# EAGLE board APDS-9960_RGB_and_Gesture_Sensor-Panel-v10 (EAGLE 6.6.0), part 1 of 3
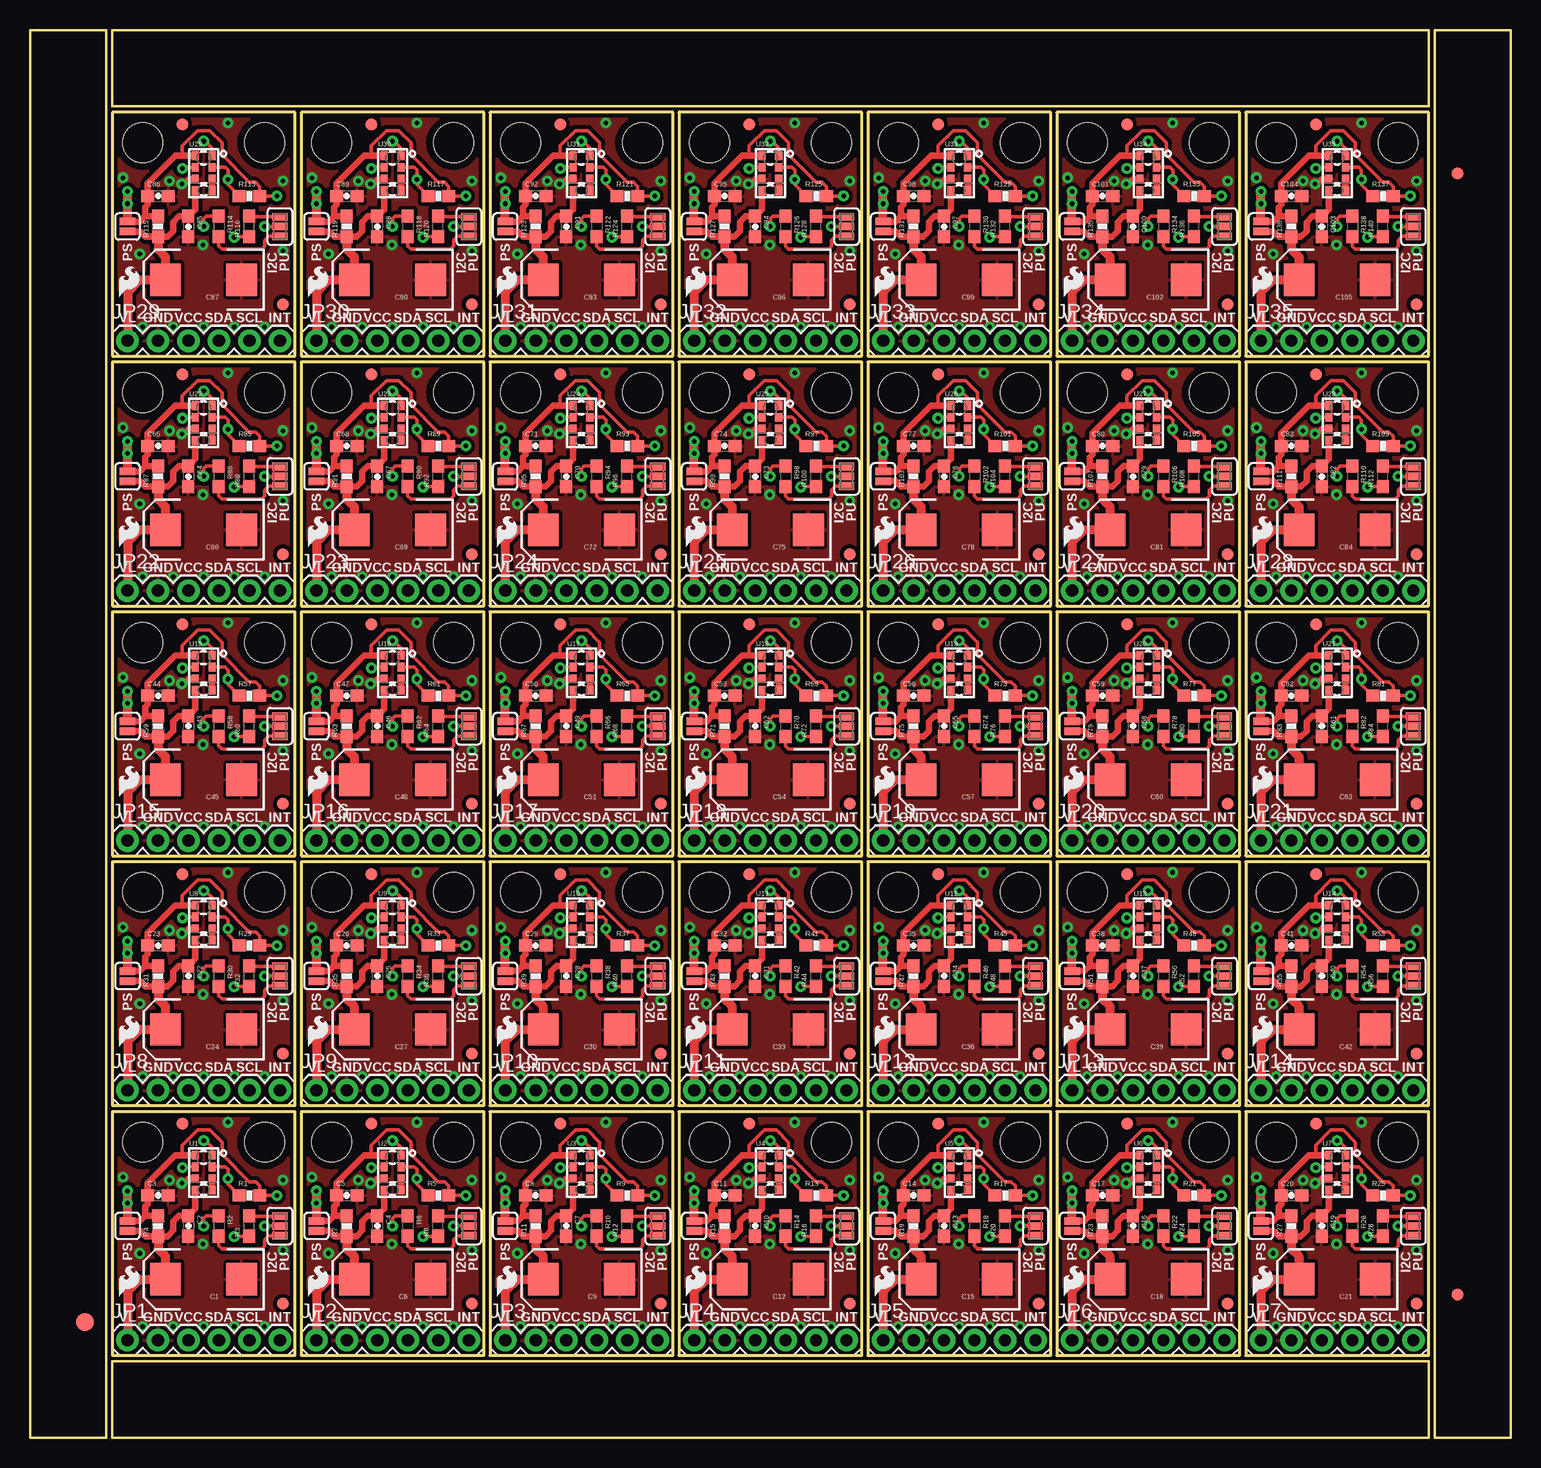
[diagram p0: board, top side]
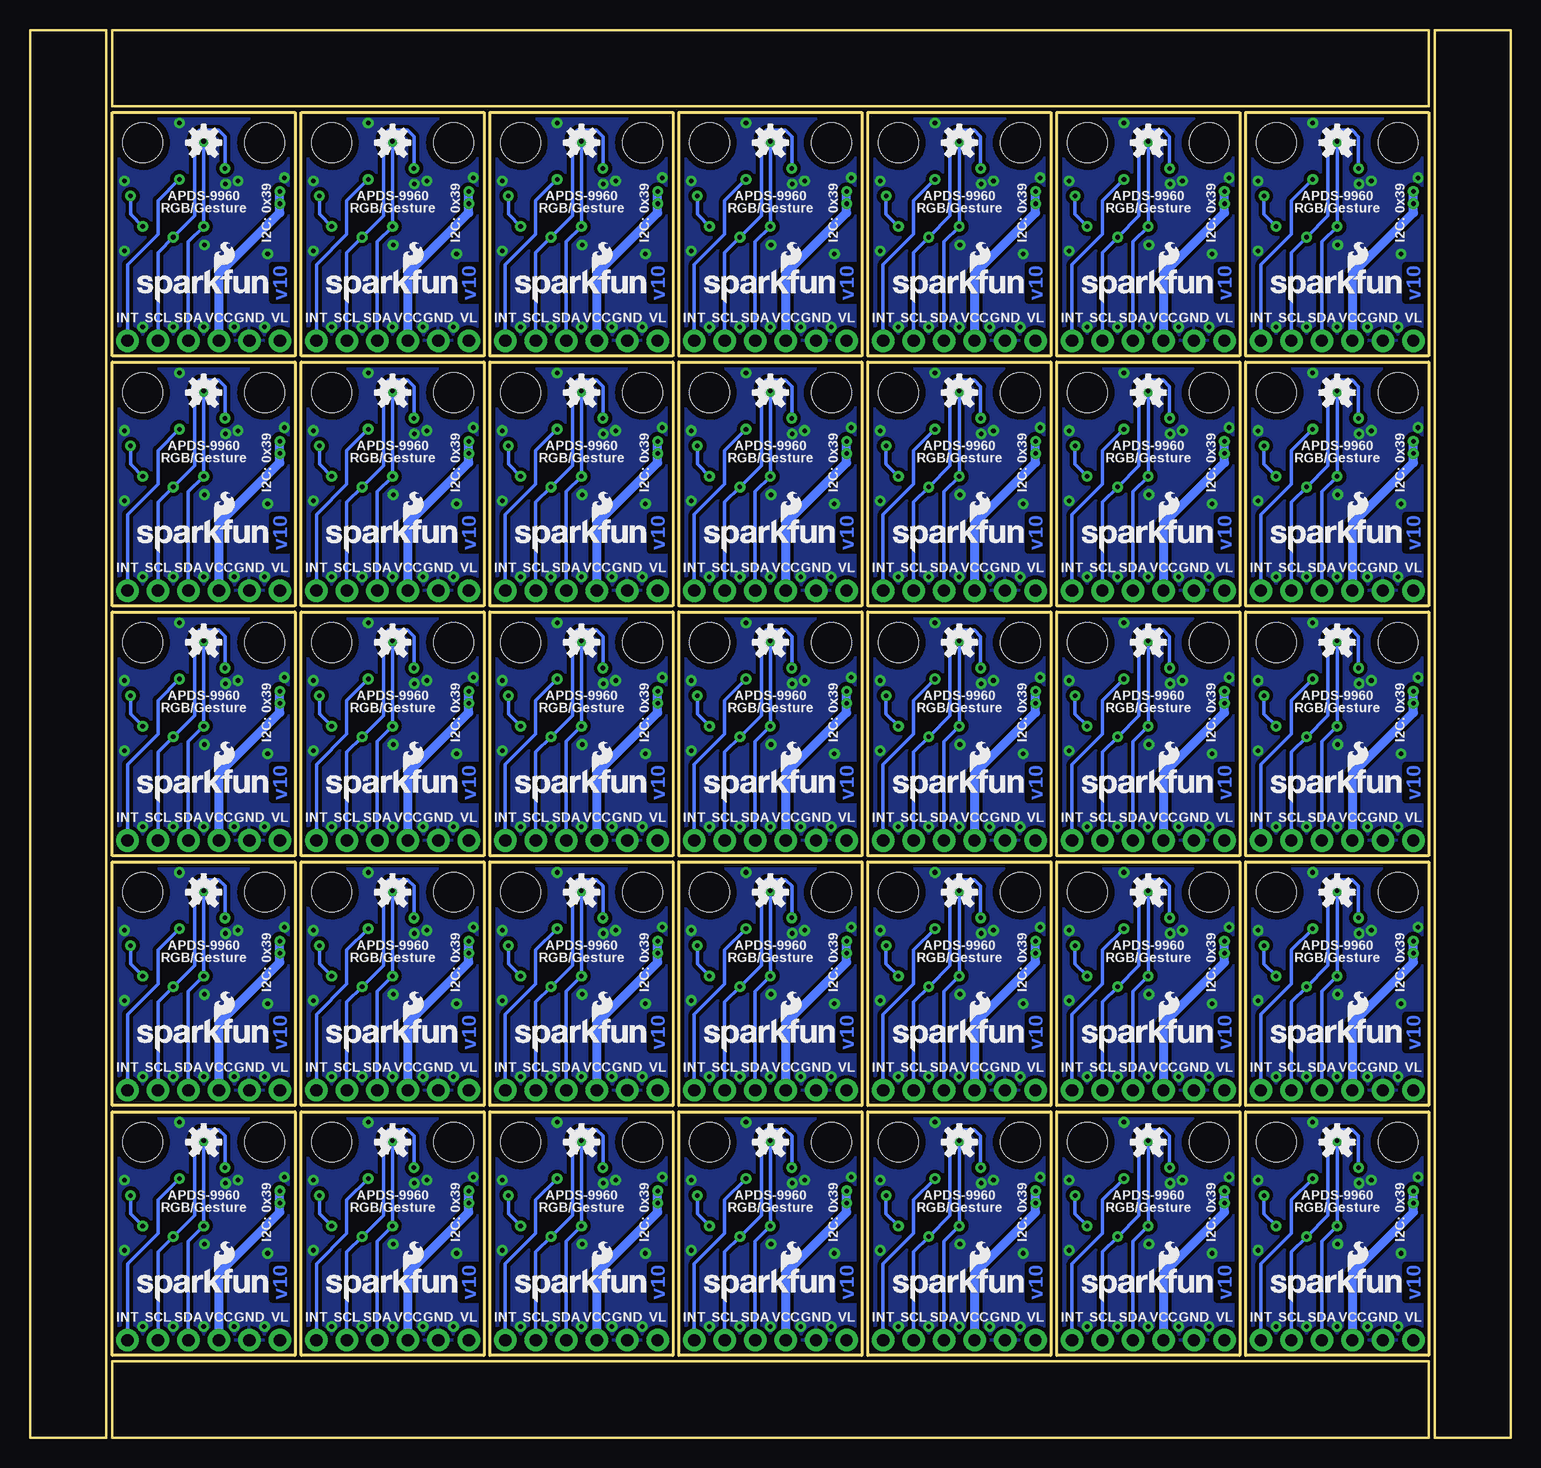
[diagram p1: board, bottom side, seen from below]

Size 123.44 x 117.35 mm. Coordinates in mm from the lower left corner, seen from the top.
Outline: 156 segments
Copper layers (1*16): Top 0.035mm / dielectric 1.5mm / Bottom 0.035mm
Design rules "SparkFun-2-layer": minimum track width 7mil, minimum drill 15mil, track to track 8mil, track to pad 8mil, pad to pad 8mil, via to via 8mil, smd to smd 8mil, copper to edge 8mil, drill to drill 8mil, minimum pad ring 12mil, minimum via ring 10mil, stop-mask expansion 4mil, vias tented up to drill 20mil, thermal gap 10mil

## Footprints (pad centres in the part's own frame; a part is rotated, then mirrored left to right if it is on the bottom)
EIA7343 = smd 2.55 x 2.7: A 3.17,0; C -3.17,0
0603-CAP = smd 1.1 x 1: 1 -0.85,0; 2 0.85,0
FIDUCIAL-1.5X3 = smd 1.5 x 1.5: 1 0,0
FIDUCIAL-1X2 = smd 1 x 1: 1 0,0
1X06 = drill 1.016 pad 1.88: 1 0,0; 2 2.54,0; 3 5.08,0; 4 7.62,0; 5 10.16,0; 6 12.7,0
0603-RES = smd 1.1 x 1: 1 -0.85,0; 2 0.85,0
0603 = smd 1.1 x 1: 1 -0.85,0; 2 0.85,0
SJ_3_PASTE1&2&3 = smd 0.635 x 1.27: 1 -0.813,0; 2 0,0; 3 0.813,0
SJ_2S = smd 0.635 x 1.27: 1 -0.412,0; 2 0.412,0
STAND-OFF = hole 3.302: 0,0
APDS-9960 = smd 0.6 x 0.72: 1 0.7,1.455; 2 0.7,0.485; 3 0.7,-0.485; 4 0.7,-1.455; 5 -0.7,-1.455; 6 -0.7,-0.485; 7 -0.7,0.485; 8 -0.7,1.455

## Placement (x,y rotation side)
C1  100uF  [EIA7343]  14.48,13.21 180 top
C2  1.0uF  [0603-CAP]  13.21,17.65 270 top
C3  1.0uF  [0603-CAP]  10.67,20.19 0 top
C4  1.0uF  [0603-CAP]  28.96,17.65 270 top
C5  1.0uF  [0603-CAP]  26.42,20.19 0 top
C6  100uF  [EIA7343]  30.23,13.21 180 top
C7  1.0uF  [0603-CAP]  44.7,17.65 270 top
C8  1.0uF  [0603-CAP]  42.16,20.19 0 top
C9  100uF  [EIA7343]  45.97,13.21 180 top
C10  1.0uF  [0603-CAP]  60.45,17.65 270 top
C11  1.0uF  [0603-CAP]  57.91,20.19 0 top
C12  100uF  [EIA7343]  61.72,13.21 180 top
C13  1.0uF  [0603-CAP]  76.2,17.65 270 top
C14  1.0uF  [0603-CAP]  73.66,20.19 0 top
C15  100uF  [EIA7343]  77.47,13.21 180 top
C16  1.0uF  [0603-CAP]  91.95,17.65 270 top
C17  1.0uF  [0603-CAP]  89.41,20.19 0 top
C18  100uF  [EIA7343]  93.22,13.21 180 top
C19  1.0uF  [0603-CAP]  107.7,17.65 270 top
C20  1.0uF  [0603-CAP]  105.16,20.19 0 top
C21  100uF  [EIA7343]  108.97,13.21 180 top
C22  1.0uF  [0603-CAP]  13.21,38.48 270 top
C23  1.0uF  [0603-CAP]  10.67,41.02 0 top
C24  100uF  [EIA7343]  14.48,34.04 180 top
C25  1.0uF  [0603-CAP]  28.96,38.48 270 top
C26  1.0uF  [0603-CAP]  26.42,41.02 0 top
C27  100uF  [EIA7343]  30.23,34.04 180 top
C28  1.0uF  [0603-CAP]  44.7,38.48 270 top
C29  1.0uF  [0603-CAP]  42.16,41.02 0 top
C30  100uF  [EIA7343]  45.97,34.04 180 top
C31  1.0uF  [0603-CAP]  60.45,38.48 270 top
C32  1.0uF  [0603-CAP]  57.91,41.02 0 top
C33  100uF  [EIA7343]  61.72,34.04 180 top
C34  1.0uF  [0603-CAP]  76.2,38.48 270 top
C35  1.0uF  [0603-CAP]  73.66,41.02 0 top
C36  100uF  [EIA7343]  77.47,34.04 180 top
C37  1.0uF  [0603-CAP]  91.95,38.48 270 top
C38  1.0uF  [0603-CAP]  89.41,41.02 0 top
C39  100uF  [EIA7343]  93.22,34.04 180 top
C40  1.0uF  [0603-CAP]  107.7,38.48 270 top
C41  1.0uF  [0603-CAP]  105.16,41.02 0 top
C42  100uF  [EIA7343]  108.97,34.04 180 top
C43  1.0uF  [0603-CAP]  13.21,59.31 270 top
C44  1.0uF  [0603-CAP]  10.67,61.85 0 top
C45  100uF  [EIA7343]  14.48,54.86 180 top
C46  1.0uF  [0603-CAP]  28.96,59.31 270 top
C47  1.0uF  [0603-CAP]  26.42,61.85 0 top
C48  100uF  [EIA7343]  30.23,54.86 180 top
C49  1.0uF  [0603-CAP]  44.7,59.31 270 top
C50  1.0uF  [0603-CAP]  42.16,61.85 0 top
C51  100uF  [EIA7343]  45.97,54.86 180 top
C52  1.0uF  [0603-CAP]  60.45,59.31 270 top
C53  1.0uF  [0603-CAP]  57.91,61.85 0 top
C54  100uF  [EIA7343]  61.72,54.86 180 top
C55  1.0uF  [0603-CAP]  76.2,59.31 270 top
C56  1.0uF  [0603-CAP]  73.66,61.85 0 top
C57  100uF  [EIA7343]  77.47,54.86 180 top
C58  1.0uF  [0603-CAP]  91.95,59.31 270 top
C59  1.0uF  [0603-CAP]  89.41,61.85 0 top
C60  100uF  [EIA7343]  93.22,54.86 180 top
C61  1.0uF  [0603-CAP]  107.7,59.31 270 top
C62  1.0uF  [0603-CAP]  105.16,61.85 0 top
C63  100uF  [EIA7343]  108.97,54.86 180 top
C64  1.0uF  [0603-CAP]  13.21,80.14 270 top
C65  1.0uF  [0603-CAP]  10.67,82.68 0 top
C66  100uF  [EIA7343]  14.48,75.69 180 top
C67  1.0uF  [0603-CAP]  28.96,80.14 270 top
C68  1.0uF  [0603-CAP]  26.42,82.68 0 top
C69  100uF  [EIA7343]  30.23,75.69 180 top
C70  1.0uF  [0603-CAP]  44.7,80.14 270 top
C71  1.0uF  [0603-CAP]  42.16,82.68 0 top
C72  100uF  [EIA7343]  45.97,75.69 180 top
C73  1.0uF  [0603-CAP]  60.45,80.14 270 top
C74  1.0uF  [0603-CAP]  57.91,82.68 0 top
C75  100uF  [EIA7343]  61.72,75.69 180 top
C76  1.0uF  [0603-CAP]  76.2,80.14 270 top
C77  1.0uF  [0603-CAP]  73.66,82.68 0 top
C78  100uF  [EIA7343]  77.47,75.69 180 top
C79  1.0uF  [0603-CAP]  91.95,80.14 270 top
C80  1.0uF  [0603-CAP]  89.41,82.68 0 top
C81  100uF  [EIA7343]  93.22,75.69 180 top
C82  1.0uF  [0603-CAP]  107.7,80.14 270 top
C83  1.0uF  [0603-CAP]  105.16,82.68 0 top
C84  100uF  [EIA7343]  108.97,75.69 180 top
C85  1.0uF  [0603-CAP]  13.21,100.97 270 top
C86  1.0uF  [0603-CAP]  10.67,103.5 0 top
C87  100uF  [EIA7343]  14.48,96.52 180 top
C88  1.0uF  [0603-CAP]  28.96,100.97 270 top
C89  1.0uF  [0603-CAP]  26.42,103.5 0 top
C90  100uF  [EIA7343]  30.23,96.52 180 top
C91  1.0uF  [0603-CAP]  44.7,100.97 270 top
C92  1.0uF  [0603-CAP]  42.16,103.5 0 top
C93  100uF  [EIA7343]  45.97,96.52 180 top
C94  1.0uF  [0603-CAP]  60.45,100.97 270 top
C95  1.0uF  [0603-CAP]  57.91,103.5 0 top
C96  100uF  [EIA7343]  61.72,96.52 180 top
C97  1.0uF  [0603-CAP]  76.2,100.97 270 top
C98  1.0uF  [0603-CAP]  73.66,103.5 0 top
C99  100uF  [EIA7343]  77.47,96.52 180 top
C100  1.0uF  [0603-CAP]  91.95,100.97 270 top
C101  1.0uF  [0603-CAP]  89.41,103.5 0 top
C102  100uF  [EIA7343]  93.22,96.52 180 top
C103  1.0uF  [0603-CAP]  107.7,100.97 270 top
C104  1.0uF  [0603-CAP]  105.16,103.5 0 top
C105  100uF  [EIA7343]  108.97,96.52 180 top
E$1  [FIDUCIAL-1.5X3]  4.57,9.65 0 top
E$4  [FIDUCIAL-1X2]  119,11.94 0 top
E$6  [FIDUCIAL-1X2]  119,105.41 180 top
FID1  FIDUCIAL1X2  [FIDUCIAL-1X2]  21.08,11.18 0 top
FID2  FIDUCIAL1X2  [FIDUCIAL-1X2]  12.7,26.16 0 top
FID3  FIDUCIAL1X2  [FIDUCIAL-1X2]  36.83,11.18 0 top
FID4  FIDUCIAL1X2  [FIDUCIAL-1X2]  28.45,26.16 0 top
FID5  FIDUCIAL1X2  [FIDUCIAL-1X2]  52.58,11.18 0 top
FID6  FIDUCIAL1X2  [FIDUCIAL-1X2]  44.2,26.16 0 top
FID7  FIDUCIAL1X2  [FIDUCIAL-1X2]  68.33,11.18 0 top
FID8  FIDUCIAL1X2  [FIDUCIAL-1X2]  59.94,26.16 0 top
FID9  FIDUCIAL1X2  [FIDUCIAL-1X2]  84.07,11.18 0 top
FID10  FIDUCIAL1X2  [FIDUCIAL-1X2]  75.69,26.16 0 top
FID11  FIDUCIAL1X2  [FIDUCIAL-1X2]  99.82,11.18 0 top
FID12  FIDUCIAL1X2  [FIDUCIAL-1X2]  91.44,26.16 0 top
FID13  FIDUCIAL1X2  [FIDUCIAL-1X2]  115.57,11.18 0 top
FID14  FIDUCIAL1X2  [FIDUCIAL-1X2]  107.19,26.16 0 top
FID15  FIDUCIAL1X2  [FIDUCIAL-1X2]  21.08,32 0 top
FID16  FIDUCIAL1X2  [FIDUCIAL-1X2]  12.7,46.99 0 top
FID17  FIDUCIAL1X2  [FIDUCIAL-1X2]  36.83,32 0 top
FID18  FIDUCIAL1X2  [FIDUCIAL-1X2]  28.45,46.99 0 top
FID19  FIDUCIAL1X2  [FIDUCIAL-1X2]  52.58,32 0 top
FID20  FIDUCIAL1X2  [FIDUCIAL-1X2]  44.2,46.99 0 top
FID21  FIDUCIAL1X2  [FIDUCIAL-1X2]  68.33,32 0 top
FID22  FIDUCIAL1X2  [FIDUCIAL-1X2]  59.94,46.99 0 top
FID23  FIDUCIAL1X2  [FIDUCIAL-1X2]  84.07,32 0 top
FID24  FIDUCIAL1X2  [FIDUCIAL-1X2]  75.69,46.99 0 top
FID25  FIDUCIAL1X2  [FIDUCIAL-1X2]  99.82,32 0 top
FID26  FIDUCIAL1X2  [FIDUCIAL-1X2]  91.44,46.99 0 top
FID27  FIDUCIAL1X2  [FIDUCIAL-1X2]  115.57,32 0 top
FID28  FIDUCIAL1X2  [FIDUCIAL-1X2]  107.19,46.99 0 top
FID29  FIDUCIAL1X2  [FIDUCIAL-1X2]  21.08,52.83 0 top
FID30  FIDUCIAL1X2  [FIDUCIAL-1X2]  12.7,67.82 0 top
FID31  FIDUCIAL1X2  [FIDUCIAL-1X2]  36.83,52.83 0 top
FID32  FIDUCIAL1X2  [FIDUCIAL-1X2]  28.45,67.82 0 top
FID33  FIDUCIAL1X2  [FIDUCIAL-1X2]  52.58,52.83 0 top
FID34  FIDUCIAL1X2  [FIDUCIAL-1X2]  44.2,67.82 0 top
FID35  FIDUCIAL1X2  [FIDUCIAL-1X2]  68.33,52.83 0 top
FID36  FIDUCIAL1X2  [FIDUCIAL-1X2]  59.94,67.82 0 top
FID37  FIDUCIAL1X2  [FIDUCIAL-1X2]  84.07,52.83 0 top
FID38  FIDUCIAL1X2  [FIDUCIAL-1X2]  75.69,67.82 0 top
FID39  FIDUCIAL1X2  [FIDUCIAL-1X2]  99.82,52.83 0 top
FID40  FIDUCIAL1X2  [FIDUCIAL-1X2]  91.44,67.82 0 top
FID41  FIDUCIAL1X2  [FIDUCIAL-1X2]  115.57,52.83 0 top
FID42  FIDUCIAL1X2  [FIDUCIAL-1X2]  107.19,67.82 0 top
FID43  FIDUCIAL1X2  [FIDUCIAL-1X2]  21.08,73.66 0 top
FID44  FIDUCIAL1X2  [FIDUCIAL-1X2]  12.7,88.65 0 top
FID45  FIDUCIAL1X2  [FIDUCIAL-1X2]  36.83,73.66 0 top
FID46  FIDUCIAL1X2  [FIDUCIAL-1X2]  28.45,88.65 0 top
FID47  FIDUCIAL1X2  [FIDUCIAL-1X2]  52.58,73.66 0 top
FID48  FIDUCIAL1X2  [FIDUCIAL-1X2]  44.2,88.65 0 top
FID49  FIDUCIAL1X2  [FIDUCIAL-1X2]  68.33,73.66 0 top
FID50  FIDUCIAL1X2  [FIDUCIAL-1X2]  59.94,88.65 0 top
FID51  FIDUCIAL1X2  [FIDUCIAL-1X2]  84.07,73.66 0 top
FID52  FIDUCIAL1X2  [FIDUCIAL-1X2]  75.69,88.65 0 top
FID53  FIDUCIAL1X2  [FIDUCIAL-1X2]  99.82,73.66 0 top
FID54  FIDUCIAL1X2  [FIDUCIAL-1X2]  91.44,88.65 0 top
FID55  FIDUCIAL1X2  [FIDUCIAL-1X2]  115.57,73.66 0 top
FID56  FIDUCIAL1X2  [FIDUCIAL-1X2]  107.19,88.65 0 top
FID57  FIDUCIAL1X2  [FIDUCIAL-1X2]  21.08,94.49 0 top
FID58  FIDUCIAL1X2  [FIDUCIAL-1X2]  12.7,109.47 0 top
FID59  FIDUCIAL1X2  [FIDUCIAL-1X2]  36.83,94.49 0 top
FID60  FIDUCIAL1X2  [FIDUCIAL-1X2]  28.45,109.47 0 top
FID61  FIDUCIAL1X2  [FIDUCIAL-1X2]  52.58,94.49 0 top
FID62  FIDUCIAL1X2  [FIDUCIAL-1X2]  44.2,109.47 0 top
FID63  FIDUCIAL1X2  [FIDUCIAL-1X2]  68.33,94.49 0 top
FID64  FIDUCIAL1X2  [FIDUCIAL-1X2]  59.94,109.47 0 top
FID65  FIDUCIAL1X2  [FIDUCIAL-1X2]  84.07,94.49 0 top
FID66  FIDUCIAL1X2  [FIDUCIAL-1X2]  75.69,109.47 0 top
FID67  FIDUCIAL1X2  [FIDUCIAL-1X2]  99.82,94.49 0 top
FID68  FIDUCIAL1X2  [FIDUCIAL-1X2]  91.44,109.47 0 top
FID69  FIDUCIAL1X2  [FIDUCIAL-1X2]  115.57,94.49 0 top
FID70  FIDUCIAL1X2  [FIDUCIAL-1X2]  107.19,109.47 0 top
JP1  [1X06]  8.13,8.13 0 top
JP2  [1X06]  23.88,8.13 0 top
JP3  [1X06]  39.62,8.13 0 top
JP4  [1X06]  55.37,8.13 0 top
JP5  [1X06]  71.12,8.13 0 top
JP6  [1X06]  86.87,8.13 0 top
JP7  [1X06]  102.62,8.13 0 top
JP8  [1X06]  8.13,28.96 0 top
JP9  [1X06]  23.88,28.96 0 top
JP10  [1X06]  39.62,28.96 0 top
JP11  [1X06]  55.37,28.96 0 top
JP12  [1X06]  71.12,28.96 0 top
JP13  [1X06]  86.87,28.96 0 top
JP14  [1X06]  102.62,28.96 0 top
JP15  [1X06]  8.13,49.78 0 top
JP16  [1X06]  23.88,49.78 0 top
JP17  [1X06]  39.62,49.78 0 top
JP18  [1X06]  55.37,49.78 0 top
JP19  [1X06]  71.12,49.78 0 top
JP20  [1X06]  86.87,49.78 0 top
JP21  [1X06]  102.62,49.78 0 top
JP22  [1X06]  8.13,70.61 0 top
JP23  [1X06]  23.88,70.61 0 top
JP24  [1X06]  39.62,70.61 0 top
JP25  [1X06]  55.37,70.61 0 top
JP26  [1X06]  71.12,70.61 0 top
JP27  [1X06]  86.87,70.61 0 top
JP28  [1X06]  102.62,70.61 0 top
JP29  [1X06]  8.13,91.44 0 top
JP30  [1X06]  23.88,91.44 0 top
JP31  [1X06]  39.62,91.44 0 top
JP32  [1X06]  55.37,91.44 0 top
JP33  [1X06]  71.12,91.44 0 top
JP34  [1X06]  86.87,91.44 0 top
JP35  [1X06]  102.62,91.44 0 top
LOGO1  SFE_LOGO_FLAME.1_INCH  [SFE_LOGO_FLAME_.1]  7.11,11.43 0 top
LOGO2  OSHW-LOGOS  [OSHW-LOGO-S]  14.48,24.64 0 bottom
LOGO3  SFE_LOGO_FLAME.1_INCH  [SFE_LOGO_FLAME_.1]  22.86,11.43 0 top
LOGO4  OSHW-LOGOS  [OSHW-LOGO-S]  30.23,24.64 0 bottom
LOGO5  SFE_LOGO_FLAME.1_INCH  [SFE_LOGO_FLAME_.1]  38.61,11.43 0 top
LOGO6  OSHW-LOGOS  [OSHW-LOGO-S]  45.97,24.64 0 bottom
LOGO7  SFE_LOGO_FLAME.1_INCH  [SFE_LOGO_FLAME_.1]  54.36,11.43 0 top
LOGO8  OSHW-LOGOS  [OSHW-LOGO-S]  61.72,24.64 0 bottom
LOGO9  SFE_LOGO_FLAME.1_INCH  [SFE_LOGO_FLAME_.1]  70.1,11.43 0 top
LOGO10  OSHW-LOGOS  [OSHW-LOGO-S]  77.47,24.64 0 bottom
LOGO11  SFE_LOGO_FLAME.1_INCH  [SFE_LOGO_FLAME_.1]  85.85,11.43 0 top
LOGO12  OSHW-LOGOS  [OSHW-LOGO-S]  93.22,24.64 0 bottom
LOGO13  SFE_LOGO_FLAME.1_INCH  [SFE_LOGO_FLAME_.1]  101.6,11.43 0 top
LOGO14  OSHW-LOGOS  [OSHW-LOGO-S]  108.97,24.64 0 bottom
LOGO15  SFE_LOGO_FLAME.1_INCH  [SFE_LOGO_FLAME_.1]  7.11,32.26 0 top
LOGO16  OSHW-LOGOS  [OSHW-LOGO-S]  14.48,45.47 0 bottom
LOGO17  SFE_LOGO_FLAME.1_INCH  [SFE_LOGO_FLAME_.1]  22.86,32.26 0 top
LOGO18  OSHW-LOGOS  [OSHW-LOGO-S]  30.23,45.47 0 bottom
LOGO19  SFE_LOGO_FLAME.1_INCH  [SFE_LOGO_FLAME_.1]  38.61,32.26 0 top
LOGO20  OSHW-LOGOS  [OSHW-LOGO-S]  45.97,45.47 0 bottom
LOGO21  SFE_LOGO_FLAME.1_INCH  [SFE_LOGO_FLAME_.1]  54.36,32.26 0 top
LOGO22  OSHW-LOGOS  [OSHW-LOGO-S]  61.72,45.47 0 bottom
LOGO23  SFE_LOGO_FLAME.1_INCH  [SFE_LOGO_FLAME_.1]  70.1,32.26 0 top
LOGO24  OSHW-LOGOS  [OSHW-LOGO-S]  77.47,45.47 0 bottom
LOGO25  SFE_LOGO_FLAME.1_INCH  [SFE_LOGO_FLAME_.1]  85.85,32.26 0 top
LOGO26  OSHW-LOGOS  [OSHW-LOGO-S]  93.22,45.47 0 bottom
LOGO27  SFE_LOGO_FLAME.1_INCH  [SFE_LOGO_FLAME_.1]  101.6,32.26 0 top
LOGO28  OSHW-LOGOS  [OSHW-LOGO-S]  108.97,45.47 0 bottom
LOGO29  SFE_LOGO_FLAME.1_INCH  [SFE_LOGO_FLAME_.1]  7.11,53.09 0 top
LOGO30  OSHW-LOGOS  [OSHW-LOGO-S]  14.48,66.29 0 bottom
LOGO31  SFE_LOGO_FLAME.1_INCH  [SFE_LOGO_FLAME_.1]  22.86,53.09 0 top
LOGO32  OSHW-LOGOS  [OSHW-LOGO-S]  30.23,66.29 0 bottom
LOGO33  SFE_LOGO_FLAME.1_INCH  [SFE_LOGO_FLAME_.1]  38.61,53.09 0 top
LOGO34  OSHW-LOGOS  [OSHW-LOGO-S]  45.97,66.29 0 bottom
LOGO35  SFE_LOGO_FLAME.1_INCH  [SFE_LOGO_FLAME_.1]  54.36,53.09 0 top
LOGO36  OSHW-LOGOS  [OSHW-LOGO-S]  61.72,66.29 0 bottom
LOGO37  SFE_LOGO_FLAME.1_INCH  [SFE_LOGO_FLAME_.1]  70.1,53.09 0 top
LOGO38  OSHW-LOGOS  [OSHW-LOGO-S]  77.47,66.29 0 bottom
LOGO39  SFE_LOGO_FLAME.1_INCH  [SFE_LOGO_FLAME_.1]  85.85,53.09 0 top
LOGO40  OSHW-LOGOS  [OSHW-LOGO-S]  93.22,66.29 0 bottom
LOGO41  SFE_LOGO_FLAME.1_INCH  [SFE_LOGO_FLAME_.1]  101.6,53.09 0 top
LOGO42  OSHW-LOGOS  [OSHW-LOGO-S]  108.97,66.29 0 bottom
LOGO43  SFE_LOGO_FLAME.1_INCH  [SFE_LOGO_FLAME_.1]  7.11,73.91 0 top
LOGO44  OSHW-LOGOS  [OSHW-LOGO-S]  14.48,87.12 0 bottom
LOGO45  SFE_LOGO_FLAME.1_INCH  [SFE_LOGO_FLAME_.1]  22.86,73.91 0 top
LOGO46  OSHW-LOGOS  [OSHW-LOGO-S]  30.23,87.12 0 bottom
LOGO47  SFE_LOGO_FLAME.1_INCH  [SFE_LOGO_FLAME_.1]  38.61,73.91 0 top
LOGO48  OSHW-LOGOS  [OSHW-LOGO-S]  45.97,87.12 0 bottom
LOGO49  SFE_LOGO_FLAME.1_INCH  [SFE_LOGO_FLAME_.1]  54.36,73.91 0 top
LOGO50  OSHW-LOGOS  [OSHW-LOGO-S]  61.72,87.12 0 bottom
LOGO51  SFE_LOGO_FLAME.1_INCH  [SFE_LOGO_FLAME_.1]  70.1,73.91 0 top
LOGO52  OSHW-LOGOS  [OSHW-LOGO-S]  77.47,87.12 0 bottom
LOGO53  SFE_LOGO_FLAME.1_INCH  [SFE_LOGO_FLAME_.1]  85.85,73.91 0 top
LOGO54  OSHW-LOGOS  [OSHW-LOGO-S]  93.22,87.12 0 bottom
LOGO55  SFE_LOGO_FLAME.1_INCH  [SFE_LOGO_FLAME_.1]  101.6,73.91 0 top
LOGO56  OSHW-LOGOS  [OSHW-LOGO-S]  108.97,87.12 0 bottom
LOGO57  SFE_LOGO_FLAME.1_INCH  [SFE_LOGO_FLAME_.1]  7.11,94.74 0 top
LOGO58  OSHW-LOGOS  [OSHW-LOGO-S]  14.48,107.95 0 bottom
LOGO59  SFE_LOGO_FLAME.1_INCH  [SFE_LOGO_FLAME_.1]  22.86,94.74 0 top
LOGO60  OSHW-LOGOS  [OSHW-LOGO-S]  30.23,107.95 0 bottom
LOGO61  SFE_LOGO_FLAME.1_INCH  [SFE_LOGO_FLAME_.1]  38.61,94.74 0 top
LOGO62  OSHW-LOGOS  [OSHW-LOGO-S]  45.97,107.95 0 bottom
LOGO63  SFE_LOGO_FLAME.1_INCH  [SFE_LOGO_FLAME_.1]  54.36,94.74 0 top
LOGO64  OSHW-LOGOS  [OSHW-LOGO-S]  61.72,107.95 0 bottom
LOGO65  SFE_LOGO_FLAME.1_INCH  [SFE_LOGO_FLAME_.1]  70.1,94.74 0 top
LOGO66  OSHW-LOGOS  [OSHW-LOGO-S]  77.47,107.95 0 bottom
LOGO67  SFE_LOGO_FLAME.1_INCH  [SFE_LOGO_FLAME_.1]  85.85,94.74 0 top
LOGO68  OSHW-LOGOS  [OSHW-LOGO-S]  93.22,107.95 0 bottom
LOGO69  SFE_LOGO_FLAME.1_INCH  [SFE_LOGO_FLAME_.1]  101.6,94.74 0 top
LOGO70  OSHW-LOGOS  [OSHW-LOGO-S]  108.97,107.95 0 bottom
R1  10k  [0603-RES]  18.29,20.19 0 top
R2  4.7k  [0603]  15.75,17.65 270 top
R3  4.7k  [0603]  18.29,17.65 90 top
R4  DNP  [0603-RES]  10.67,17.65 90 top
R5  10k  [0603-RES]  34.04,20.19 0 top
R6  4.7k  [0603]  31.5,17.65 270 top
R7  DNP  [0603-RES]  26.42,17.65 90 top
R8  4.7k  [0603]  34.04,17.65 90 top
R9  10k  [0603-RES]  49.78,20.19 0 top
R10  4.7k  [0603]  47.24,17.65 270 top
R11  DNP  [0603-RES]  42.16,17.65 90 top
R12  4.7k  [0603]  49.78,17.65 90 top
R13  10k  [0603-RES]  65.53,20.19 0 top
R14  4.7k  [0603]  62.99,17.65 270 top
R15  DNP  [0603-RES]  57.91,17.65 90 top
R16  4.7k  [0603]  65.53,17.65 90 top
R17  10k  [0603-RES]  81.28,20.19 0 top
R18  4.7k  [0603]  78.74,17.65 270 top
R19  DNP  [0603-RES]  73.66,17.65 90 top
R20  4.7k  [0603]  81.28,17.65 90 top
R21  10k  [0603-RES]  97.03,20.19 0 top
R22  4.7k  [0603]  94.49,17.65 270 top
R23  DNP  [0603-RES]  89.41,17.65 90 top
R24  4.7k  [0603]  97.03,17.65 90 top
R25  10k  [0603-RES]  112.78,20.19 0 top
R26  4.7k  [0603]  110.24,17.65 270 top
R27  DNP  [0603-RES]  105.16,17.65 90 top
R28  4.7k  [0603]  112.78,17.65 90 top
R29  10k  [0603-RES]  18.29,41.02 0 top
R30  4.7k  [0603]  15.75,38.48 270 top
R31  DNP  [0603-RES]  10.67,38.48 90 top
R32  4.7k  [0603]  18.29,38.48 90 top
R33  10k  [0603-RES]  34.04,41.02 0 top
R34  4.7k  [0603]  31.5,38.48 270 top
R35  DNP  [0603-RES]  26.42,38.48 90 top
R36  4.7k  [0603]  34.04,38.48 90 top
R37  10k  [0603-RES]  49.78,41.02 0 top
R38  4.7k  [0603]  47.24,38.48 270 top
R39  DNP  [0603-RES]  42.16,38.48 90 top
R40  4.7k  [0603]  49.78,38.48 90 top
R41  10k  [0603-RES]  65.53,41.02 0 top
R42  4.7k  [0603]  62.99,38.48 270 top
R43  DNP  [0603-RES]  57.91,38.48 90 top
R44  4.7k  [0603]  65.53,38.48 90 top
R45  10k  [0603-RES]  81.28,41.02 0 top
R46  4.7k  [0603]  78.74,38.48 270 top
R47  DNP  [0603-RES]  73.66,38.48 90 top
R48  4.7k  [0603]  81.28,38.48 90 top
R49  10k  [0603-RES]  97.03,41.02 0 top
R50  4.7k  [0603]  94.49,38.48 270 top
R51  DNP  [0603-RES]  89.41,38.48 90 top
R52  4.7k  [0603]  97.03,38.48 90 top
R53  10k  [0603-RES]  112.78,41.02 0 top
R54  4.7k  [0603]  110.24,38.48 270 top
R55  DNP  [0603-RES]  105.16,38.48 90 top
R56  4.7k  [0603]  112.78,38.48 90 top
R57  10k  [0603-RES]  18.29,61.85 0 top
R58  4.7k  [0603]  15.75,59.31 270 top
R59  DNP  [0603-RES]  10.67,59.31 90 top
R60  4.7k  [0603]  18.29,59.31 90 top
R61  10k  [0603-RES]  34.04,61.85 0 top
R62  4.7k  [0603]  31.5,59.31 270 top
R63  DNP  [0603-RES]  26.42,59.31 90 top
R64  4.7k  [0603]  34.04,59.31 90 top
R65  10k  [0603-RES]  49.78,61.85 0 top
R66  4.7k  [0603]  47.24,59.31 270 top
R67  DNP  [0603-RES]  42.16,59.31 90 top
R68  4.7k  [0603]  49.78,59.31 90 top
R69  10k  [0603-RES]  65.53,61.85 0 top
R70  4.7k  [0603]  62.99,59.31 270 top
R71  DNP  [0603-RES]  57.91,59.31 90 top
R72  4.7k  [0603]  65.53,59.31 90 top
R73  10k  [0603-RES]  81.28,61.85 0 top
R74  4.7k  [0603]  78.74,59.31 270 top
R75  DNP  [0603-RES]  73.66,59.31 90 top
R76  4.7k  [0603]  81.28,59.31 90 top
R77  10k  [0603-RES]  97.03,61.85 0 top
R78  4.7k  [0603]  94.49,59.31 270 top
R79  DNP  [0603-RES]  89.41,59.31 90 top
R80  4.7k  [0603]  97.03,59.31 90 top
R81  10k  [0603-RES]  112.78,61.85 0 top
R82  4.7k  [0603]  110.24,59.31 270 top
R83  DNP  [0603-RES]  105.16,59.31 90 top
R84  4.7k  [0603]  112.78,59.31 90 top
R85  10k  [0603-RES]  18.29,82.68 0 top
R86  4.7k  [0603]  15.75,80.14 270 top
R87  DNP  [0603-RES]  10.67,80.14 90 top
R88  4.7k  [0603]  18.29,80.14 90 top
R89  10k  [0603-RES]  34.04,82.68 0 top
R90  4.7k  [0603]  31.5,80.14 270 top
R91  DNP  [0603-RES]  26.42,80.14 90 top
R92  4.7k  [0603]  34.04,80.14 90 top
R93  10k  [0603-RES]  49.78,82.68 0 top
R94  4.7k  [0603]  47.24,80.14 270 top
R95  DNP  [0603-RES]  42.16,80.14 90 top
R96  4.7k  [0603]  49.78,80.14 90 top
R97  10k  [0603-RES]  65.53,82.68 0 top
R98  4.7k  [0603]  62.99,80.14 270 top
R99  DNP  [0603-RES]  57.91,80.14 90 top
R100  4.7k  [0603]  65.53,80.14 90 top
R101  10k  [0603-RES]  81.28,82.68 0 top
R102  4.7k  [0603]  78.74,80.14 270 top
R103  DNP  [0603-RES]  73.66,80.14 90 top
R104  4.7k  [0603]  81.28,80.14 90 top
R105  10k  [0603-RES]  97.03,82.68 0 top
R106  4.7k  [0603]  94.49,80.14 270 top
R107  DNP  [0603-RES]  89.41,80.14 90 top
R108  4.7k  [0603]  97.03,80.14 90 top
R109  10k  [0603-RES]  112.78,82.68 0 top
R110  4.7k  [0603]  110.24,80.14 270 top
R111  DNP  [0603-RES]  105.16,80.14 90 top
R112  4.7k  [0603]  112.78,80.14 90 top
R113  10k  [0603-RES]  18.29,103.5 0 top
R114  4.7k  [0603]  15.75,100.97 270 top
R115  DNP  [0603-RES]  10.67,100.97 90 top
R116  4.7k  [0603]  18.29,100.97 90 top
R117  10k  [0603-RES]  34.04,103.5 0 top
R118  4.7k  [0603]  31.5,100.97 270 top
R119  DNP  [0603-RES]  26.42,100.97 90 top
R120  4.7k  [0603]  34.04,100.97 90 top
R121  10k  [0603-RES]  49.78,103.5 0 top
R122  4.7k  [0603]  47.24,100.97 270 top
R123  DNP  [0603-RES]  42.16,100.97 90 top
R124  4.7k  [0603]  49.78,100.97 90 top
R125  10k  [0603-RES]  65.53,103.5 0 top
R126  4.7k  [0603]  62.99,100.97 270 top
R127  DNP  [0603-RES]  57.91,100.97 90 top
R128  4.7k  [0603]  65.53,100.97 90 top
R129  10k  [0603-RES]  81.28,103.5 0 top
R130  4.7k  [0603]  78.74,100.97 270 top
R131  DNP  [0603-RES]  73.66,100.97 90 top
R132  4.7k  [0603]  81.28,100.97 90 top
R133  10k  [0603-RES]  97.03,103.5 0 top
R134  4.7k  [0603]  94.49,100.97 270 top
R135  DNP  [0603-RES]  89.41,100.97 90 top
R136  4.7k  [0603]  97.03,100.97 90 top
R137  10k  [0603-RES]  112.78,103.5 0 top
R138  4.7k  [0603]  110.24,100.97 270 top
R139  DNP  [0603-RES]  105.16,100.97 90 top
R140  4.7k  [0603]  112.78,100.97 90 top
SJ1  [SJ_3_PASTE1&2&3]  20.83,17.65 270 top
SJ2  SOLDERJUMPERNC  [SJ_2S]  8.13,17.65 90 top
SJ3  [SJ_3_PASTE1&2&3]  36.58,17.65 270 top
SJ4  SOLDERJUMPERNC  [SJ_2S]  23.88,17.65 90 top
SJ5  [SJ_3_PASTE1&2&3]  52.32,17.65 270 top
SJ6  SOLDERJUMPERNC  [SJ_2S]  39.62,17.65 90 top
SJ7  [SJ_3_PASTE1&2&3]  68.07,17.65 270 top
SJ8  SOLDERJUMPERNC  [SJ_2S]  55.37,17.65 90 top
SJ9  [SJ_3_PASTE1&2&3]  83.82,17.65 270 top
SJ10  SOLDERJUMPERNC  [SJ_2S]  71.12,17.65 90 top
SJ11  [SJ_3_PASTE1&2&3]  99.57,17.65 270 top
SJ12  SOLDERJUMPERNC  [SJ_2S]  86.87,17.65 90 top
SJ13  [SJ_3_PASTE1&2&3]  115.32,17.65 270 top
SJ14  SOLDERJUMPERNC  [SJ_2S]  102.62,17.65 90 top
SJ15  [SJ_3_PASTE1&2&3]  20.83,38.48 270 top
SJ16  SOLDERJUMPERNC  [SJ_2S]  8.13,38.48 90 top
SJ17  [SJ_3_PASTE1&2&3]  36.58,38.48 270 top
SJ18  SOLDERJUMPERNC  [SJ_2S]  23.88,38.48 90 top
SJ19  [SJ_3_PASTE1&2&3]  52.32,38.48 270 top
SJ20  SOLDERJUMPERNC  [SJ_2S]  39.62,38.48 90 top
SJ21  [SJ_3_PASTE1&2&3]  68.07,38.48 270 top
SJ22  SOLDERJUMPERNC  [SJ_2S]  55.37,38.48 90 top
SJ23  [SJ_3_PASTE1&2&3]  83.82,38.48 270 top
SJ24  SOLDERJUMPERNC  [SJ_2S]  71.12,38.48 90 top
SJ25  [SJ_3_PASTE1&2&3]  99.57,38.48 270 top
SJ26  SOLDERJUMPERNC  [SJ_2S]  86.87,38.48 90 top
SJ27  [SJ_3_PASTE1&2&3]  115.32,38.48 270 top
SJ28  SOLDERJUMPERNC  [SJ_2S]  102.62,38.48 90 top
SJ29  [SJ_3_PASTE1&2&3]  20.83,59.31 270 top
SJ30  SOLDERJUMPERNC  [SJ_2S]  8.13,59.31 90 top
SJ31  [SJ_3_PASTE1&2&3]  36.58,59.31 270 top
SJ32  SOLDERJUMPERNC  [SJ_2S]  23.88,59.31 90 top
SJ33  [SJ_3_PASTE1&2&3]  52.32,59.31 270 top
SJ34  SOLDERJUMPERNC  [SJ_2S]  39.62,59.31 90 top
SJ35  [SJ_3_PASTE1&2&3]  68.07,59.31 270 top
SJ36  SOLDERJUMPERNC  [SJ_2S]  55.37,59.31 90 top
SJ37  [SJ_3_PASTE1&2&3]  83.82,59.31 270 top
SJ38  SOLDERJUMPERNC  [SJ_2S]  71.12,59.31 90 top
SJ39  [SJ_3_PASTE1&2&3]  99.57,59.31 270 top
SJ40  SOLDERJUMPERNC  [SJ_2S]  86.87,59.31 90 top
SJ41  [SJ_3_PASTE1&2&3]  115.32,59.31 270 top
SJ42  SOLDERJUMPERNC  [SJ_2S]  102.62,59.31 90 top
SJ43  [SJ_3_PASTE1&2&3]  20.83,80.14 270 top
SJ44  SOLDERJUMPERNC  [SJ_2S]  8.13,80.14 90 top
SJ45  [SJ_3_PASTE1&2&3]  36.58,80.14 270 top
SJ46  SOLDERJUMPERNC  [SJ_2S]  23.88,80.14 90 top
SJ47  [SJ_3_PASTE1&2&3]  52.32,80.14 270 top
SJ48  SOLDERJUMPERNC  [SJ_2S]  39.62,80.14 90 top
SJ49  [SJ_3_PASTE1&2&3]  68.07,80.14 270 top
SJ50  SOLDERJUMPERNC  [SJ_2S]  55.37,80.14 90 top
SJ51  [SJ_3_PASTE1&2&3]  83.82,80.14 270 top
SJ52  SOLDERJUMPERNC  [SJ_2S]  71.12,80.14 90 top
SJ53  [SJ_3_PASTE1&2&3]  99.57,80.14 270 top
SJ54  SOLDERJUMPERNC  [SJ_2S]  86.87,80.14 90 top
SJ55  [SJ_3_PASTE1&2&3]  115.32,80.14 270 top
SJ56  SOLDERJUMPERNC  [SJ_2S]  102.62,80.14 90 top
SJ57  [SJ_3_PASTE1&2&3]  20.83,100.97 270 top
SJ58  SOLDERJUMPERNC  [SJ_2S]  8.13,100.97 90 top
SJ59  [SJ_3_PASTE1&2&3]  36.58,100.97 270 top
SJ60  SOLDERJUMPERNC  [SJ_2S]  23.88,100.97 90 top
SJ61  [SJ_3_PASTE1&2&3]  52.32,100.97 270 top
SJ62  SOLDERJUMPERNC  [SJ_2S]  39.62,100.97 90 top
SJ63  [SJ_3_PASTE1&2&3]  68.07,100.97 270 top
SJ64  SOLDERJUMPERNC  [SJ_2S]  55.37,100.97 90 top
SJ65  [SJ_3_PASTE1&2&3]  83.82,100.97 270 top
SJ66  SOLDERJUMPERNC  [SJ_2S]  71.12,100.97 90 top
SJ67  [SJ_3_PASTE1&2&3]  99.57,100.97 270 top
SJ68  SOLDERJUMPERNC  [SJ_2S]  86.87,100.97 90 top
SJ69  [SJ_3_PASTE1&2&3]  115.32,100.97 270 top
SJ70  SOLDERJUMPERNC  [SJ_2S]  102.62,100.97 90 top
STANDOFF1  STAND-OFF  [STAND-OFF]  9.4,24.64 0 top
STANDOFF2  STAND-OFF  [STAND-OFF]  19.56,24.64 0 top
STANDOFF3  STAND-OFF  [STAND-OFF]  25.15,24.64 0 top
STANDOFF4  STAND-OFF  [STAND-OFF]  35.31,24.64 0 top
STANDOFF5  STAND-OFF  [STAND-OFF]  40.89,24.64 0 top
STANDOFF6  STAND-OFF  [STAND-OFF]  51.05,24.64 0 top
STANDOFF7  STAND-OFF  [STAND-OFF]  56.64,24.64 0 top
STANDOFF8  STAND-OFF  [STAND-OFF]  66.8,24.64 0 top
STANDOFF9  STAND-OFF  [STAND-OFF]  72.39,24.64 0 top
STANDOFF10  STAND-OFF  [STAND-OFF]  82.55,24.64 0 top
STANDOFF11  STAND-OFF  [STAND-OFF]  88.14,24.64 0 top
STANDOFF12  STAND-OFF  [STAND-OFF]  98.3,24.64 0 top
STANDOFF13  STAND-OFF  [STAND-OFF]  103.89,24.64 0 top
STANDOFF14  STAND-OFF  [STAND-OFF]  114.05,24.64 0 top
STANDOFF15  STAND-OFF  [STAND-OFF]  9.4,45.47 0 top
STANDOFF16  STAND-OFF  [STAND-OFF]  19.56,45.47 0 top
STANDOFF17  STAND-OFF  [STAND-OFF]  25.15,45.47 0 top
STANDOFF18  STAND-OFF  [STAND-OFF]  35.31,45.47 0 top
STANDOFF19  STAND-OFF  [STAND-OFF]  40.89,45.47 0 top
STANDOFF20  STAND-OFF  [STAND-OFF]  51.05,45.47 0 top
STANDOFF21  STAND-OFF  [STAND-OFF]  56.64,45.47 0 top
STANDOFF22  STAND-OFF  [STAND-OFF]  66.8,45.47 0 top
STANDOFF23  STAND-OFF  [STAND-OFF]  72.39,45.47 0 top
STANDOFF24  STAND-OFF  [STAND-OFF]  82.55,45.47 0 top
STANDOFF25  STAND-OFF  [STAND-OFF]  88.14,45.47 0 top
STANDOFF26  STAND-OFF  [STAND-OFF]  98.3,45.47 0 top
STANDOFF27  STAND-OFF  [STAND-OFF]  103.89,45.47 0 top
STANDOFF28  STAND-OFF  [STAND-OFF]  114.05,45.47 0 top
STANDOFF29  STAND-OFF  [STAND-OFF]  9.4,66.29 0 top
STANDOFF30  STAND-OFF  [STAND-OFF]  19.56,66.29 0 top
STANDOFF31  STAND-OFF  [STAND-OFF]  25.15,66.29 0 top
STANDOFF32  STAND-OFF  [STAND-OFF]  35.31,66.29 0 top
STANDOFF33  STAND-OFF  [STAND-OFF]  40.89,66.29 0 top
STANDOFF34  STAND-OFF  [STAND-OFF]  51.05,66.29 0 top
STANDOFF35  STAND-OFF  [STAND-OFF]  56.64,66.29 0 top
STANDOFF36  STAND-OFF  [STAND-OFF]  66.8,66.29 0 top
STANDOFF37  STAND-OFF  [STAND-OFF]  72.39,66.29 0 top
STANDOFF38  STAND-OFF  [STAND-OFF]  82.55,66.29 0 top
STANDOFF39  STAND-OFF  [STAND-OFF]  88.14,66.29 0 top
STANDOFF40  STAND-OFF  [STAND-OFF]  98.3,66.29 0 top
STANDOFF41  STAND-OFF  [STAND-OFF]  103.89,66.29 0 top
STANDOFF42  STAND-OFF  [STAND-OFF]  114.05,66.29 0 top
STANDOFF43  STAND-OFF  [STAND-OFF]  9.4,87.12 0 top
STANDOFF44  STAND-OFF  [STAND-OFF]  19.56,87.12 0 top
STANDOFF45  STAND-OFF  [STAND-OFF]  25.15,87.12 0 top
STANDOFF46  STAND-OFF  [STAND-OFF]  35.31,87.12 0 top
STANDOFF47  STAND-OFF  [STAND-OFF]  40.89,87.12 0 top
STANDOFF48  STAND-OFF  [STAND-OFF]  51.05,87.12 0 top
STANDOFF49  STAND-OFF  [STAND-OFF]  56.64,87.12 0 top
STANDOFF50  STAND-OFF  [STAND-OFF]  66.8,87.12 0 top
STANDOFF51  STAND-OFF  [STAND-OFF]  72.39,87.12 0 top
STANDOFF52  STAND-OFF  [STAND-OFF]  82.55,87.12 0 top
STANDOFF53  STAND-OFF  [STAND-OFF]  88.14,87.12 0 top
STANDOFF54  STAND-OFF  [STAND-OFF]  98.3,87.12 0 top
STANDOFF55  STAND-OFF  [STAND-OFF]  103.89,87.12 0 top
STANDOFF56  STAND-OFF  [STAND-OFF]  114.05,87.12 0 top
STANDOFF57  STAND-OFF  [STAND-OFF]  9.4,107.95 0 top
STANDOFF58  STAND-OFF  [STAND-OFF]  19.56,107.95 0 top
STANDOFF59  STAND-OFF  [STAND-OFF]  25.15,107.95 0 top
STANDOFF60  STAND-OFF  [STAND-OFF]  35.31,107.95 0 top
STANDOFF61  STAND-OFF  [STAND-OFF]  40.89,107.95 0 top
STANDOFF62  STAND-OFF  [STAND-OFF]  51.05,107.95 0 top
STANDOFF63  STAND-OFF  [STAND-OFF]  56.64,107.95 0 top
STANDOFF64  STAND-OFF  [STAND-OFF]  66.8,107.95 0 top
STANDOFF65  STAND-OFF  [STAND-OFF]  72.39,107.95 0 top
STANDOFF66  STAND-OFF  [STAND-OFF]  82.55,107.95 0 top
STANDOFF67  STAND-OFF  [STAND-OFF]  88.14,107.95 0 top
STANDOFF68  STAND-OFF  [STAND-OFF]  98.3,107.95 0 top
STANDOFF69  STAND-OFF  [STAND-OFF]  103.89,107.95 0 top
STANDOFF70  STAND-OFF  [STAND-OFF]  114.05,107.95 0 top
U1  APDS-9960  [APDS-9960]  14.48,22.1 0 top
U2  APDS-9960  [APDS-9960]  30.23,22.1 0 top
U3  APDS-9960  [APDS-9960]  45.97,22.1 0 top
U4  APDS-9960  [APDS-9960]  61.72,22.1 0 top
U5  APDS-9960  [APDS-9960]  77.47,22.1 0 top
U6  APDS-9960  [APDS-9960]  93.22,22.1 0 top
U7  APDS-9960  [APDS-9960]  108.97,22.1 0 top
U8  APDS-9960  [APDS-9960]  14.48,42.93 0 top
U9  APDS-9960  [APDS-9960]  30.23,42.93 0 top
U10  APDS-9960  [APDS-9960]  45.97,42.93 0 top
U11  APDS-9960  [APDS-9960]  61.72,42.93 0 top
U12  APDS-9960  [APDS-9960]  77.47,42.93 0 top
U13  APDS-9960  [APDS-9960]  93.22,42.93 0 top
U14  APDS-9960  [APDS-9960]  108.97,42.93 0 top
U15  APDS-9960  [APDS-9960]  14.48,63.75 0 top
U16  APDS-9960  [APDS-9960]  30.23,63.75 0 top
U17  APDS-9960  [APDS-9960]  45.97,63.75 0 top
U18  APDS-9960  [APDS-9960]  61.72,63.75 0 top
U19  APDS-9960  [APDS-9960]  77.47,63.75 0 top
U20  APDS-9960  [APDS-9960]  93.22,63.75 0 top
U21  APDS-9960  [APDS-9960]  108.97,63.75 0 top
U22  APDS-9960  [APDS-9960]  14.48,84.58 0 top
U23  APDS-9960  [APDS-9960]  30.23,84.58 0 top
U24  APDS-9960  [APDS-9960]  45.97,84.58 0 top
U25  APDS-9960  [APDS-9960]  61.72,84.58 0 top
U26  APDS-9960  [APDS-9960]  77.47,84.58 0 top
U27  APDS-9960  [APDS-9960]  93.22,84.58 0 top
U28  APDS-9960  [APDS-9960]  108.97,84.58 0 top
U29  APDS-9960  [APDS-9960]  14.48,105.41 0 top
U30  APDS-9960  [APDS-9960]  30.23,105.41 0 top
U31  APDS-9960  [APDS-9960]  45.97,105.41 0 top
U32  APDS-9960  [APDS-9960]  61.72,105.41 0 top
U33  APDS-9960  [APDS-9960]  77.47,105.41 0 top
U34  APDS-9960  [APDS-9960]  93.22,105.41 0 top
U35  APDS-9960  [APDS-9960]  108.97,105.41 0 top
U$1  SFE_LOGO_NAME_FLAME.1_INCH  [SFE_LOGO_NAME_FLAME_.1]  20.45,11.18 0 bottom
U$2  SFE_LOGO_NAME_FLAME.1_INCH  [SFE_LOGO_NAME_FLAME_.1]  36.2,11.18 0 bottom
U$3  SFE_LOGO_NAME_FLAME.1_INCH  [SFE_LOGO_NAME_FLAME_.1]  51.94,11.18 0 bottom
U$4  SFE_LOGO_NAME_FLAME.1_INCH  [SFE_LOGO_NAME_FLAME_.1]  67.69,11.18 0 bottom
U$5  SFE_LOGO_NAME_FLAME.1_INCH  [SFE_LOGO_NAME_FLAME_.1]  83.44,11.18 0 bottom
U$6  SFE_LOGO_NAME_FLAME.1_INCH  [SFE_LOGO_NAME_FLAME_.1]  99.19,11.18 0 bottom
U$7  SFE_LOGO_NAME_FLAME.1_INCH  [SFE_LOGO_NAME_FLAME_.1]  114.94,11.18 0 bottom
U$8  SFE_LOGO_NAME_FLAME.1_INCH  [SFE_LOGO_NAME_FLAME_.1]  20.45,32 0 bottom
U$9  SFE_LOGO_NAME_FLAME.1_INCH  [SFE_LOGO_NAME_FLAME_.1]  36.2,32 0 bottom
U$10  SFE_LOGO_NAME_FLAME.1_INCH  [SFE_LOGO_NAME_FLAME_.1]  51.94,32 0 bottom
U$11  SFE_LOGO_NAME_FLAME.1_INCH  [SFE_LOGO_NAME_FLAME_.1]  67.69,32 0 bottom
U$12  SFE_LOGO_NAME_FLAME.1_INCH  [SFE_LOGO_NAME_FLAME_.1]  83.44,32 0 bottom
U$13  SFE_LOGO_NAME_FLAME.1_INCH  [SFE_LOGO_NAME_FLAME_.1]  99.19,32 0 bottom
U$14  SFE_LOGO_NAME_FLAME.1_INCH  [SFE_LOGO_NAME_FLAME_.1]  114.94,32 0 bottom
U$15  SFE_LOGO_NAME_FLAME.1_INCH  [SFE_LOGO_NAME_FLAME_.1]  20.45,52.83 0 bottom
U$16  SFE_LOGO_NAME_FLAME.1_INCH  [SFE_LOGO_NAME_FLAME_.1]  36.2,52.83 0 bottom
U$17  SFE_LOGO_NAME_FLAME.1_INCH  [SFE_LOGO_NAME_FLAME_.1]  51.94,52.83 0 bottom
U$18  SFE_LOGO_NAME_FLAME.1_INCH  [SFE_LOGO_NAME_FLAME_.1]  67.69,52.83 0 bottom
U$19  SFE_LOGO_NAME_FLAME.1_INCH  [SFE_LOGO_NAME_FLAME_.1]  83.44,52.83 0 bottom
U$20  SFE_LOGO_NAME_FLAME.1_INCH  [SFE_LOGO_NAME_FLAME_.1]  99.19,52.83 0 bottom
U$21  SFE_LOGO_NAME_FLAME.1_INCH  [SFE_LOGO_NAME_FLAME_.1]  114.94,52.83 0 bottom
U$22  SFE_LOGO_NAME_FLAME.1_INCH  [SFE_LOGO_NAME_FLAME_.1]  20.45,73.66 0 bottom
U$23  SFE_LOGO_NAME_FLAME.1_INCH  [SFE_LOGO_NAME_FLAME_.1]  36.2,73.66 0 bottom
U$24  SFE_LOGO_NAME_FLAME.1_INCH  [SFE_LOGO_NAME_FLAME_.1]  51.94,73.66 0 bottom
U$25  SFE_LOGO_NAME_FLAME.1_INCH  [SFE_LOGO_NAME_FLAME_.1]  67.69,73.66 0 bottom
U$26  SFE_LOGO_NAME_FLAME.1_INCH  [SFE_LOGO_NAME_FLAME_.1]  83.44,73.66 0 bottom
U$27  SFE_LOGO_NAME_FLAME.1_INCH  [SFE_LOGO_NAME_FLAME_.1]  99.19,73.66 0 bottom
U$28  SFE_LOGO_NAME_FLAME.1_INCH  [SFE_LOGO_NAME_FLAME_.1]  114.94,73.66 0 bottom
U$29  SFE_LOGO_NAME_FLAME.1_INCH  [SFE_LOGO_NAME_FLAME_.1]  20.45,94.49 0 bottom
U$30  SFE_LOGO_NAME_FLAME.1_INCH  [SFE_LOGO_NAME_FLAME_.1]  36.2,94.49 0 bottom
U$31  SFE_LOGO_NAME_FLAME.1_INCH  [SFE_LOGO_NAME_FLAME_.1]  51.94,94.49 0 bottom
U$32  SFE_LOGO_NAME_FLAME.1_INCH  [SFE_LOGO_NAME_FLAME_.1]  67.69,94.49 0 bottom
U$33  SFE_LOGO_NAME_FLAME.1_INCH  [SFE_LOGO_NAME_FLAME_.1]  83.44,94.49 0 bottom
U$34  SFE_LOGO_NAME_FLAME.1_INCH  [SFE_LOGO_NAME_FLAME_.1]  99.19,94.49 0 bottom
U$35  SFE_LOGO_NAME_FLAME.1_INCH  [SFE_LOGO_NAME_FLAME_.1]  114.94,94.49 0 bottom

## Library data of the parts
C1 C6 C9 C12 C15 C18 C21 C24 C27 C30 C33 C36 C39 C42 C45 C48 C51 C54 C57 C60 C63 C66 C69 C72 C75 C78 C81 C84 C87 C90 C93 C96 C99 C102 C105 = SparkFun-Capacitors; PROD_ID: CAP-07890
C2-C5 C7 C8 C10 C11 C13 C14 C16 C17 C19 C20 C22 C23 C25 C26 C28 C29 C31 C32 C34 C35 C37 C38 C40 C41 C43 C44 C46 C47 C49 C50 C52 C53 C55 C56 C58 C59 C61 C62 C64 C65 C67 C68 C70 C71 C73 C74 C76 C77 C79 C80 C82 C83 C85 C86 C88 C89 C91 C92 C94 C95 C97 C98 C100 C101 C103 C104 = SparkFun-Capacitors; PROD_ID: CAP-00868
E$1 SJ2 SJ4 SJ6 SJ8 SJ10 SJ12 SJ14 SJ16 SJ18 SJ20 SJ22 SJ24 SJ26 SJ28 SJ30 SJ32 SJ34 SJ36 SJ38 SJ40 SJ42 SJ44 SJ46 SJ48 SJ50 SJ52 SJ54 SJ56 SJ58 SJ60 SJ62 SJ64 SJ66 SJ68 SJ70 = SparkFun-Retired
E$4 E$6 FID1-FID70 LOGO1-LOGO70 U$1-U$35 = SparkFun-Aesthetics
JP1-JP35 = SparkFun-Connectors
R1 R5 R9 R13 R17 R21 R25 R29 R33 R37 R41 R45 R49 R53 R57 R61 R65 R69 R73 R77 R81 R85 R89 R93 R97 R101 R105 R109 R113 R117 R121 R125 R129 R133 R137 = SparkFun-Resistors; PROD_ID: RES-00824
R2 R3 R6 R8 R10 R12 R14 R16 R18 R20 R22 R24 R26 R28 R30 R32 R34 R36 R38 R40 R42 R44 R46 R48 R50 R52 R54 R56 R58 R60 R62 R64 R66 R68 R70 R72 R74 R76 R78 R80 R82 R84 R86 R88 R90 R92 R94 R96 R98 R100 R102 R104 R106 R108 R110 R112 R114 R116 R118 R120 R122 R124 R126 R128 R130 R132 R134 R136 R138 R140 = SparkFun-Resistors; PROD_ID: RES-07857
R4 R7 R11 R15 R19 R23 R27 R31 R35 R39 R43 R47 R51 R55 R59 R63 R67 R71 R75 R79 R83 R87 R91 R95 R99 R103 R107 R111 R115 R119 R123 R127 R131 R135 R139 = SparkFun-Resistors
SJ1 SJ3 SJ5 SJ7 SJ9 SJ11 SJ13 SJ15 SJ17 SJ19 SJ21 SJ23 SJ25 SJ27 SJ29 SJ31 SJ33 SJ35 SJ37 SJ39 SJ41 SJ43 SJ45 SJ47 SJ49 SJ51 SJ53 SJ55 SJ57 SJ59 SJ61 SJ63 SJ65 SJ67 SJ69 = SparkFun-Passives
STANDOFF1-STANDOFF70 = SparkFun-Electromechanical
U1-U35 = SparkFun-Sensors; PROD_ID: SEN-12005

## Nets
GND: C1.C C2.2 C3.2 JP1.2 U1.6
GND1: C4.2 C5.2 C6.C JP2.2 U2.6
GND2: C7.2 C8.2 C9.C JP3.2 U3.6
GND3: C10.2 C11.2 C12.C JP4.2 U4.6
GND4: C13.2 C14.2 C15.C JP5.2 U5.6
GND5: C16.2 C17.2 C18.C JP6.2 U6.6
GND6: C19.2 C20.2 C21.C JP7.2 U7.6
GND7: C22.2 C23.2 C24.C JP8.2 U8.6
GND8: C25.2 C26.2 C27.C JP9.2 U9.6
GND9: C28.2 C29.2 C30.C JP10.2 U10.6
GND10: C31.2 C32.2 C33.C JP11.2 U11.6
GND11: C34.2 C35.2 C36.C JP12.2 U12.6
GND12: C37.2 C38.2 C39.C JP13.2 U13.6
GND13: C40.2 C41.2 C42.C JP14.2 U14.6
GND14: C43.2 C44.2 C45.C JP15.2 U15.6
GND15: C46.2 C47.2 C48.C JP16.2 U16.6
GND16: C49.2 C50.2 C51.C JP17.2 U17.6
GND17: C52.2 C53.2 C54.C JP18.2 U18.6
GND18: C55.2 C56.2 C57.C JP19.2 U19.6
GND19: C58.2 C59.2 C60.C JP20.2 U20.6
GND20: C61.2 C62.2 C63.C JP21.2 U21.6
GND21: C64.2 C65.2 C66.C JP22.2 U22.6
GND22: C67.2 C68.2 C69.C JP23.2 U23.6
GND23: C70.2 C71.2 C72.C JP24.2 U24.6
GND24: C73.2 C74.2 C75.C JP25.2 U25.6
GND25: C76.2 C77.2 C78.C JP26.2 U26.6
GND26: C79.2 C80.2 C81.C JP27.2 U27.6
GND27: C82.2 C83.2 C84.C JP28.2 U28.6
GND28: C85.2 C86.2 C87.C JP29.2 U29.6
GND29: C88.2 C89.2 C90.C JP30.2 U30.6
GND30: C91.2 C92.2 C93.C JP31.2 U31.6
GND31: C94.2 C95.2 C96.C JP32.2 U32.6
GND32: C97.2 C98.2 C99.C JP33.2 U33.6
GND33: C100.2 C101.2 C102.C JP34.2 U34.6
GND34: C103.2 C104.2 C105.C JP35.2 U35.6
INT: JP1.6 R1.1 U1.2
INT1: JP2.6 R5.1 U2.2
INT2: JP3.6 R9.1 U3.2
INT3: JP4.6 R13.1 U4.2
INT4: JP5.6 R17.1 U5.2
INT5: JP6.6 R21.1 U6.2
INT6: JP7.6 R25.1 U7.2
INT7: JP8.6 R29.1 U8.2
INT8: JP9.6 R33.1 U9.2
INT9: JP10.6 R37.1 U10.2
INT10: JP11.6 R41.1 U11.2
INT11: JP12.6 R45.1 U12.2
INT12: JP13.6 R49.1 U13.2
INT13: JP14.6 R53.1 U14.2
INT14: JP15.6 R57.1 U15.2
INT15: JP16.6 R61.1 U16.2
INT16: JP17.6 R65.1 U17.2
INT17: JP18.6 R69.1 U18.2
INT18: JP19.6 R73.1 U19.2
INT19: JP20.6 R77.1 U20.2
INT20: JP21.6 R81.1 U21.2
INT21: JP22.6 R85.1 U22.2
INT22: JP23.6 R89.1 U23.2
INT23: JP24.6 R93.1 U24.2
INT24: JP25.6 R97.1 U25.2
INT25: JP26.6 R101.1 U26.2
INT26: JP27.6 R105.1 U27.2
INT27: JP28.6 R109.1 U28.2
INT28: JP29.6 R113.1 U29.2
INT29: JP30.6 R117.1 U30.2
INT30: JP31.6 R121.1 U31.2
INT31: JP32.6 R125.1 U32.2
INT32: JP33.6 R129.1 U33.2
INT33: JP34.6 R133.1 U34.2
INT34: JP35.6 R137.1 U35.2
N$1: R2.2 SJ1.3
N$2: R3.2 SJ1.1
N$4: U1.3 U1.4
N$5: R6.2 SJ3.3
N$6: R8.2 SJ3.1
N$7: U2.3 U2.4
N$8: R10.2 SJ5.3
N$9: R12.2 SJ5.1
N$10: U3.3 U3.4
N$11: R14.2 SJ7.3
N$12: R16.2 SJ7.1
N$13: U4.3 U4.4
N$14: R18.2 SJ9.3
N$15: R20.2 SJ9.1
N$16: U5.3 U5.4
N$17: R22.2 SJ11.3
N$18: R24.2 SJ11.1
N$19: U6.3 U6.4
N$20: R26.2 SJ13.3
N$21: R28.2 SJ13.1
N$22: U7.3 U7.4
N$23: R30.2 SJ15.3
N$24: R32.2 SJ15.1
N$25: U8.3 U8.4
N$26: R34.2 SJ17.3
N$27: R36.2 SJ17.1
N$28: U9.3 U9.4
N$29: R38.2 SJ19.3
N$30: R40.2 SJ19.1
N$31: U10.3 U10.4
N$32: R42.2 SJ21.3
N$33: R44.2 SJ21.1
N$34: U11.3 U11.4
N$35: R46.2 SJ23.3
N$36: R48.2 SJ23.1
N$37: U12.3 U12.4
N$38: R50.2 SJ25.3
N$39: R52.2 SJ25.1
N$40: U13.3 U13.4
N$41: R54.2 SJ27.3
N$42: R56.2 SJ27.1
N$43: U14.3 U14.4
N$44: R58.2 SJ29.3
N$45: R60.2 SJ29.1
N$46: U15.3 U15.4
N$47: R62.2 SJ31.3
N$48: R64.2 SJ31.1
N$49: U16.3 U16.4
N$50: R66.2 SJ33.3
N$51: R68.2 SJ33.1
N$52: U17.3 U17.4
N$53: R70.2 SJ35.3
N$54: R72.2 SJ35.1
N$55: U18.3 U18.4
N$56: R74.2 SJ37.3
N$57: R76.2 SJ37.1
N$58: U19.3 U19.4
N$59: R78.2 SJ39.3
N$60: R80.2 SJ39.1
N$61: U20.3 U20.4
N$62: R82.2 SJ41.3
N$63: R84.2 SJ41.1
N$64: U21.3 U21.4
N$65: R86.2 SJ43.3
N$66: R88.2 SJ43.1
N$67: U22.3 U22.4
N$68: R90.2 SJ45.3
N$69: R92.2 SJ45.1
N$70: U23.3 U23.4
N$71: R94.2 SJ47.3
N$72: R96.2 SJ47.1
N$73: U24.3 U24.4
N$74: R98.2 SJ49.3
N$75: R100.2 SJ49.1
N$76: U25.3 U25.4
N$77: R102.2 SJ51.3
N$78: R104.2 SJ51.1
N$79: U26.3 U26.4
N$80: R106.2 SJ53.3
N$81: R108.2 SJ53.1
N$82: U27.3 U27.4
N$83: R110.2 SJ55.3
N$84: R112.2 SJ55.1
N$85: U28.3 U28.4
N$86: R114.2 SJ57.3
N$87: R116.2 SJ57.1
N$88: U29.3 U29.4
N$89: R118.2 SJ59.3
N$90: R120.2 SJ59.1
N$91: U30.3 U30.4
N$92: R122.2 SJ61.3
N$93: R124.2 SJ61.1
N$94: U31.3 U31.4
N$95: R126.2 SJ63.3
N$96: R128.2 SJ63.1
N$97: U32.3 U32.4
N$98: R130.2 SJ65.3
N$99: R132.2 SJ65.1
N$100: U33.3 U33.4
N$101: R134.2 SJ67.3
N$102: R136.2 SJ67.1
N$103: U34.3 U34.4
N$104: R138.2 SJ69.3
N$105: R140.2 SJ69.1
N$106: U35.3 U35.4
SCL: JP1.5 R3.1 U1.7
SCL1: JP2.5 R8.1 U2.7
SCL2: JP3.5 R12.1 U3.7
SCL3: JP4.5 R16.1 U4.7
SCL4: JP5.5 R20.1 U5.7
SCL5: JP6.5 R24.1 U6.7
SCL6: JP7.5 R28.1 U7.7
SCL7: JP8.5 R32.1 U8.7
SCL8: JP9.5 R36.1 U9.7
SCL9: JP10.5 R40.1 U10.7
SCL10: JP11.5 R44.1 U11.7
SCL11: JP12.5 R48.1 U12.7
SCL12: JP13.5 R52.1 U13.7
SCL13: JP14.5 R56.1 U14.7
SCL14: JP15.5 R60.1 U15.7
SCL15: JP16.5 R64.1 U16.7
SCL16: JP17.5 R68.1 U17.7
SCL17: JP18.5 R72.1 U18.7
SCL18: JP19.5 R76.1 U19.7
SCL19: JP20.5 R80.1 U20.7
SCL20: JP21.5 R84.1 U21.7
SCL21: JP22.5 R88.1 U22.7
SCL22: JP23.5 R92.1 U23.7
SCL23: JP24.5 R96.1 U24.7
SCL24: JP25.5 R100.1 U25.7
SCL25: JP26.5 R104.1 U26.7
SCL26: JP27.5 R108.1 U27.7
SCL27: JP28.5 R112.1 U28.7
SCL28: JP29.5 R116.1 U29.7
SCL29: JP30.5 R120.1 U30.7
SCL30: JP31.5 R124.1 U31.7
SCL31: JP32.5 R128.1 U32.7
SCL32: JP33.5 R132.1 U33.7
SCL33: JP34.5 R136.1 U34.7
SCL34: JP35.5 R140.1 U35.7
SDA: JP1.4 R2.1 U1.1
SDA1: JP2.4 R6.1 U2.1
SDA2: JP3.4 R10.1 U3.1
SDA3: JP4.4 R14.1 U4.1
SDA4: JP5.4 R18.1 U5.1
SDA5: JP6.4 R22.1 U6.1
SDA6: JP7.4 R26.1 U7.1
SDA7: JP8.4 R30.1 U8.1
SDA8: JP9.4 R34.1 U9.1
SDA9: JP10.4 R38.1 U10.1
SDA10: JP11.4 R42.1 U11.1
SDA11: JP12.4 R46.1 U12.1
SDA12: JP13.4 R50.1 U13.1
SDA13: JP14.4 R54.1 U14.1
SDA14: JP15.4 R58.1 U15.1
SDA15: JP16.4 R62.1 U16.1
SDA16: JP17.4 R66.1 U17.1
SDA17: JP18.4 R70.1 U18.1
SDA18: JP19.4 R74.1 U19.1
SDA19: JP20.4 R78.1 U20.1
SDA20: JP21.4 R82.1 U21.1
SDA21: JP22.4 R86.1 U22.1
SDA22: JP23.4 R90.1 U23.1
SDA23: JP24.4 R94.1 U24.1
SDA24: JP25.4 R98.1 U25.1
SDA25: JP26.4 R102.1 U26.1
SDA26: JP27.4 R106.1 U27.1
SDA27: JP28.4 R110.1 U28.1
SDA28: JP29.4 R114.1 U29.1
SDA29: JP30.4 R118.1 U30.1
SDA30: JP31.4 R122.1 U31.1
SDA31: JP32.4 R126.1 U32.1
SDA32: JP33.4 R130.1 U33.1
SDA33: JP34.4 R134.1 U34.1
SDA34: JP35.4 R138.1 U35.1
VCC: C3.1 JP1.3 R1.2 R4.2 SJ1.2 SJ2.2 U1.8
VCC1: C5.1 JP2.3 R5.2 R7.2 SJ3.2 SJ4.2 U2.8
VCC2: C8.1 JP3.3 R9.2 R11.2 SJ5.2 SJ6.2 U3.8
VCC3: C11.1 JP4.3 R13.2 R15.2 SJ7.2 SJ8.2 U4.8
VCC4: C14.1 JP5.3 R17.2 R19.2 SJ9.2 SJ10.2 U5.8
VCC5: C17.1 JP6.3 R21.2 R23.2 SJ11.2 SJ12.2 U6.8
VCC6: C20.1 JP7.3 R25.2 R27.2 SJ13.2 SJ14.2 U7.8
VCC7: C23.1 JP8.3 R29.2 R31.2 SJ15.2 SJ16.2 U8.8
VCC8: C26.1 JP9.3 R33.2 R35.2 SJ17.2 SJ18.2 U9.8
VCC9: C29.1 JP10.3 R37.2 R39.2 SJ19.2 SJ20.2 U10.8
VCC10: C32.1 JP11.3 R41.2 R43.2 SJ21.2 SJ22.2 U11.8
VCC11: C35.1 JP12.3 R45.2 R47.2 SJ23.2 SJ24.2 U12.8
VCC12: C38.1 JP13.3 R49.2 R51.2 SJ25.2 SJ26.2 U13.8
VCC13: C41.1 JP14.3 R53.2 R55.2 SJ27.2 SJ28.2 U14.8
VCC14: C44.1 JP15.3 R57.2 R59.2 SJ29.2 SJ30.2 U15.8
VCC15: C47.1 JP16.3 R61.2 R63.2 SJ31.2 SJ32.2 U16.8
VCC16: C50.1 JP17.3 R65.2 R67.2 SJ33.2 SJ34.2 U17.8
VCC17: C53.1 JP18.3 R69.2 R71.2 SJ35.2 SJ36.2 U18.8
VCC18: C56.1 JP19.3 R73.2 R75.2 SJ37.2 SJ38.2 U19.8
VCC19: C59.1 JP20.3 R77.2 R79.2 SJ39.2 SJ40.2 U20.8
VCC20: C62.1 JP21.3 R81.2 R83.2 SJ41.2 SJ42.2 U21.8
VCC21: C65.1 JP22.3 R85.2 R87.2 SJ43.2 SJ44.2 U22.8
VCC22: C68.1 JP23.3 R89.2 R91.2 SJ45.2 SJ46.2 U23.8
VCC23: C71.1 JP24.3 R93.2 R95.2 SJ47.2 SJ48.2 U24.8
VCC24: C74.1 JP25.3 R97.2 R99.2 SJ49.2 SJ50.2 U25.8
VCC25: C77.1 JP26.3 R101.2 R103.2 SJ51.2 SJ52.2 U26.8
VCC26: C80.1 JP27.3 R105.2 R107.2 SJ53.2 SJ54.2 U27.8
VCC27: C83.1 JP28.3 R109.2 R111.2 SJ55.2 SJ56.2 U28.8
VCC28: C86.1 JP29.3 R113.2 R115.2 SJ57.2 SJ58.2 U29.8
VCC29: C89.1 JP30.3 R117.2 R119.2 SJ59.2 SJ60.2 U30.8
VCC30: C92.1 JP31.3 R121.2 R123.2 SJ61.2 SJ62.2 U31.8
VCC31: C95.1 JP32.3 R125.2 R127.2 SJ63.2 SJ64.2 U32.8
VCC32: C98.1 JP33.3 R129.2 R131.2 SJ65.2 SJ66.2 U33.8
VCC33: C101.1 JP34.3 R133.2 R135.2 SJ67.2 SJ68.2 U34.8
VCC34: C104.1 JP35.3 R137.2 R139.2 SJ69.2 SJ70.2 U35.8
VL: C1.A C2.1 JP1.1 R4.1 SJ2.1 U1.5
VL1: C4.1 C6.A JP2.1 R7.1 SJ4.1 U2.5
VL2: C7.1 C9.A JP3.1 R11.1 SJ6.1 U3.5
VL3: C10.1 C12.A JP4.1 R15.1 SJ8.1 U4.5
VL4: C13.1 C15.A JP5.1 R19.1 SJ10.1 U5.5
VL5: C16.1 C18.A JP6.1 R23.1 SJ12.1 U6.5
VL6: C19.1 C21.A JP7.1 R27.1 SJ14.1 U7.5
VL7: C22.1 C24.A JP8.1 R31.1 SJ16.1 U8.5
VL8: C25.1 C27.A JP9.1 R35.1 SJ18.1 U9.5
VL9: C28.1 C30.A JP10.1 R39.1 SJ20.1 U10.5
VL10: C31.1 C33.A JP11.1 R43.1 SJ22.1 U11.5
VL11: C34.1 C36.A JP12.1 R47.1 SJ24.1 U12.5
VL12: C37.1 C39.A JP13.1 R51.1 SJ26.1 U13.5
VL13: C40.1 C42.A JP14.1 R55.1 SJ28.1 U14.5
VL14: C43.1 C45.A JP15.1 R59.1 SJ30.1 U15.5
VL15: C46.1 C48.A JP16.1 R63.1 SJ32.1 U16.5
VL16: C49.1 C51.A JP17.1 R67.1 SJ34.1 U17.5
VL17: C52.1 C54.A JP18.1 R71.1 SJ36.1 U18.5
VL18: C55.1 C57.A JP19.1 R75.1 SJ38.1 U19.5
VL19: C58.1 C60.A JP20.1 R79.1 SJ40.1 U20.5
VL20: C61.1 C63.A JP21.1 R83.1 SJ42.1 U21.5
VL21: C64.1 C66.A JP22.1 R87.1 SJ44.1 U22.5
VL22: C67.1 C69.A JP23.1 R91.1 SJ46.1 U23.5
VL23: C70.1 C72.A JP24.1 R95.1 SJ48.1 U24.5
VL24: C73.1 C75.A JP25.1 R99.1 SJ50.1 U25.5
VL25: C76.1 C78.A JP26.1 R103.1 SJ52.1 U26.5
VL26: C79.1 C81.A JP27.1 R107.1 SJ54.1 U27.5
VL27: C82.1 C84.A JP28.1 R111.1 SJ56.1 U28.5
VL28: C85.1 C87.A JP29.1 R115.1 SJ58.1 U29.5
VL29: C88.1 C90.A JP30.1 R119.1 SJ60.1 U30.5
VL30: C91.1 C93.A JP31.1 R123.1 SJ62.1 U31.5
VL31: C94.1 C96.A JP32.1 R127.1 SJ64.1 U32.5
VL32: C97.1 C99.A JP33.1 R131.1 SJ66.1 U33.5
VL33: C100.1 C102.A JP34.1 R135.1 SJ68.1 U34.5
VL34: C103.1 C105.A JP35.1 R139.1 SJ70.1 U35.5

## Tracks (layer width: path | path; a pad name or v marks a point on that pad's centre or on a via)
GND  (via drill 0.38)
  Top 0.559: 13.77,21.61 13.26,21.61 13.26,21.59 12.93,21.26
  other vias: 12.65,21.21 11.63,21.46 14.43,16.13 14.48,9.27 19.56,9.27 21.08,15.62 17.02,9.27 9.4,9.27 11.94,9.27 9.14,15.37 16.51,26.29 21.08,21.46 7.75,21.72
  pour Top (isolate 0.305): 6.86,27.18 22.1,27.18 22.1,6.86 6.86,6.86
  pour Bottom (isolate 0.305): 6.86,27.18 22.1,27.18 22.1,6.86 6.86,6.86
GND1  (via drill 0.38)
  Top 0.559: 29.52,21.61 29.01,21.61 29.01,21.59 28.68,21.26
  other vias: 28.4,21.21 27.38,21.46 30.18,16.13 30.23,9.27 35.31,9.27 36.83,15.62 32.77,9.27 25.15,9.27 27.69,9.27 24.89,15.37 32.26,26.29 36.83,21.46 23.5,21.72
  pour Top (isolate 0.305): 22.61,27.18 37.85,27.18 37.85,6.86 22.61,6.86
  pour Bottom (isolate 0.305): 22.61,27.18 37.85,27.18 37.85,6.86 22.61,6.86
GND2  (via drill 0.38)
  Top 0.559: U3.6 44.76,21.61 44.76,21.59 44.42,21.26
  other vias: 44.15,21.21 43.13,21.46 45.92,16.13 45.97,9.27 51.05,9.27 52.58,15.62 48.51,9.27 40.89,9.27 43.43,9.27 40.64,15.37 48.01,26.29 52.58,21.46 39.24,21.72
  pour Top (isolate 0.305): 38.35,27.18 53.59,27.18 53.59,6.86 38.35,6.86
  pour Bottom (isolate 0.305): 38.35,27.18 53.59,27.18 53.59,6.86 38.35,6.86
GND3  (via drill 0.38)
  Top 0.559: U4.6 60.5,21.61 60.5,21.59 60.17,21.26
  other vias: 59.89,21.21 58.88,21.46 61.67,16.13 61.72,9.27 66.8,9.27 68.33,15.62 64.26,9.27 56.64,9.27 59.18,9.27 56.39,15.37 63.75,26.29 68.33,21.46 54.99,21.72
  pour Top (isolate 0.305): 54.1,27.18 69.34,27.18 69.34,6.86 54.1,6.86
  pour Bottom (isolate 0.305): 54.1,27.18 69.34,27.18 69.34,6.86 54.1,6.86
GND4  (via drill 0.38)
  Top 0.559: U5.6 76.25,21.61 76.25,21.59 75.92,21.26
  other vias: 75.64,21.21 74.63,21.46 77.42,16.13 77.47,9.27 82.55,9.27 84.07,15.62 80.01,9.27 72.39,9.27 74.93,9.27 72.14,15.37 79.5,26.29 84.07,21.46 70.74,21.72
  pour Top (isolate 0.305): 69.85,27.18 85.09,27.18 85.09,6.86 69.85,6.86
  pour Bottom (isolate 0.305): 69.85,27.18 85.09,27.18 85.09,6.86 69.85,6.86
GND5  (via drill 0.38)
  Top 0.559: 92.51,21.61 92,21.61 92,21.59 91.67,21.26
  other vias: 91.39,21.21 90.37,21.46 93.17,16.13 93.22,9.27 98.3,9.27 99.82,15.62 95.76,9.27 88.14,9.27 90.68,9.27 87.88,15.37 95.25,26.29 99.82,21.46 86.49,21.72
  pour Top (isolate 0.305): 85.6,27.18 100.84,27.18 100.84,6.86 85.6,6.86
  pour Bottom (isolate 0.305): 85.6,27.18 100.84,27.18 100.84,6.86 85.6,6.86
GND6  (via drill 0.38)
  Top 0.559: 108.25,21.61 107.75,21.61 107.75,21.59 107.42,21.26
  other vias: 107.14,21.21 106.12,21.46 108.92,16.13 108.97,9.27 114.05,9.27 115.57,15.62 111.51,9.27 103.89,9.27 106.43,9.27 103.63,15.37 111,26.29 115.57,21.46 102.23,21.72
  pour Top (isolate 0.305): 101.35,27.18 116.59,27.18 116.59,6.86 101.35,6.86
  pour Bottom (isolate 0.305): 101.35,27.18 116.59,27.18 116.59,6.86 101.35,6.86
GND7  (via drill 0.38)
  Top 0.559: 13.77,42.44 13.26,42.44 13.26,42.42 12.93,42.09
  other vias: 12.65,42.04 11.63,42.29 14.43,36.96 14.48,30.1 19.56,30.1 21.08,36.45 17.02,30.1 9.4,30.1 11.94,30.1 9.14,36.2 16.51,47.12 21.08,42.29 7.75,42.55
  pour Top (isolate 0.305): 6.86,48.01 22.1,48.01 22.1,27.69 6.86,27.69
  pour Bottom (isolate 0.305): 6.86,48.01 22.1,48.01 22.1,27.69 6.86,27.69
GND8  (via drill 0.38)
  Top 0.559: 29.52,42.44 29.01,42.44 29.01,42.42 28.68,42.09
  other vias: 28.4,42.04 27.38,42.29 30.18,36.96 30.23,30.1 35.31,30.1 36.83,36.45 32.77,30.1 25.15,30.1 27.69,30.1 24.89,36.2 32.26,47.12 36.83,42.29 23.5,42.55
  pour Top (isolate 0.305): 22.61,48.01 37.85,48.01 37.85,27.69 22.61,27.69
  pour Bottom (isolate 0.305): 22.61,48.01 37.85,48.01 37.85,27.69 22.61,27.69
GND9  (via drill 0.38)
  Top 0.559: U10.6 44.76,42.44 44.76,42.42 44.42,42.09
  other vias: 44.15,42.04 43.13,42.29 45.92,36.96 45.97,30.1 51.05,30.1 52.58,36.45 48.51,30.1 40.89,30.1 43.43,30.1 40.64,36.2 48.01,47.12 52.58,42.29 39.24,42.55
  pour Top (isolate 0.305): 38.35,48.01 53.59,48.01 53.59,27.69 38.35,27.69
  pour Bottom (isolate 0.305): 38.35,48.01 53.59,48.01 53.59,27.69 38.35,27.69
GND10  (via drill 0.38)
  Top 0.559: U11.6 60.5,42.44 60.5,42.42 60.17,42.09
  other vias: 59.89,42.04 58.88,42.29 61.67,36.96 61.72,30.1 66.8,30.1 68.33,36.45 64.26,30.1 56.64,30.1 59.18,30.1 56.39,36.2 63.75,47.12 68.33,42.29 54.99,42.55
  pour Top (isolate 0.305): 54.1,48.01 69.34,48.01 69.34,27.69 54.1,27.69
  pour Bottom (isolate 0.305): 54.1,48.01 69.34,48.01 69.34,27.69 54.1,27.69
GND11  (via drill 0.38)
  Top 0.559: U12.6 76.25,42.44 76.25,42.42 75.92,42.09
  other vias: 75.64,42.04 74.63,42.29 77.42,36.96 77.47,30.1 82.55,30.1 84.07,36.45 80.01,30.1 72.39,30.1 74.93,30.1 72.14,36.2 79.5,47.12 84.07,42.29 70.74,42.55
  pour Top (isolate 0.305): 69.85,48.01 85.09,48.01 85.09,27.69 69.85,27.69
  pour Bottom (isolate 0.305): 69.85,48.01 85.09,48.01 85.09,27.69 69.85,27.69
GND12  (via drill 0.38)
  Top 0.559: 92.51,42.44 92,42.44 92,42.42 91.67,42.09
  other vias: 91.39,42.04 90.37,42.29 93.17,36.96 93.22,30.1 98.3,30.1 99.82,36.45 95.76,30.1 88.14,30.1 90.68,30.1 87.88,36.2 95.25,47.12 99.82,42.29 86.49,42.55
  pour Top (isolate 0.305): 85.6,48.01 100.84,48.01 100.84,27.69 85.6,27.69
  pour Bottom (isolate 0.305): 85.6,48.01 100.84,48.01 100.84,27.69 85.6,27.69
GND13  (via drill 0.38)
  Top 0.559: 108.25,42.44 107.75,42.44 107.75,42.42 107.42,42.09
  other vias: 107.14,42.04 106.12,42.29 108.92,36.96 108.97,30.1 114.05,30.1 115.57,36.45 111.51,30.1 103.89,30.1 106.43,30.1 103.63,36.2 111,47.12 115.57,42.29 102.23,42.55
  pour Top (isolate 0.305): 101.35,48.01 116.59,48.01 116.59,27.69 101.35,27.69
  pour Bottom (isolate 0.305): 101.35,48.01 116.59,48.01 116.59,27.69 101.35,27.69
GND14  (via drill 0.38)
  Top 0.559: 13.77,63.27 13.26,63.27 13.26,63.25 12.93,62.92
  other vias: 12.65,62.87 11.63,63.12 14.43,57.78 14.48,50.93 19.56,50.93 21.08,57.28 17.02,50.93 9.4,50.93 11.94,50.93 9.14,57.02 16.51,67.94 21.08,63.12 7.75,63.37
  pour Top (isolate 0.305): 6.86,68.83 22.1,68.83 22.1,48.51 6.86,48.51
  pour Bottom (isolate 0.305): 6.86,68.83 22.1,68.83 22.1,48.51 6.86,48.51
GND15  (via drill 0.38)
  Top 0.559: 29.52,63.27 29.01,63.27 29.01,63.25 28.68,62.92

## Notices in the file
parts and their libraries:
SparkFun-Aesthetics: Licensing: Creative Commons ShareAlike 4.0 International - https://creativecommons.org/licenses/by-sa/4.0
